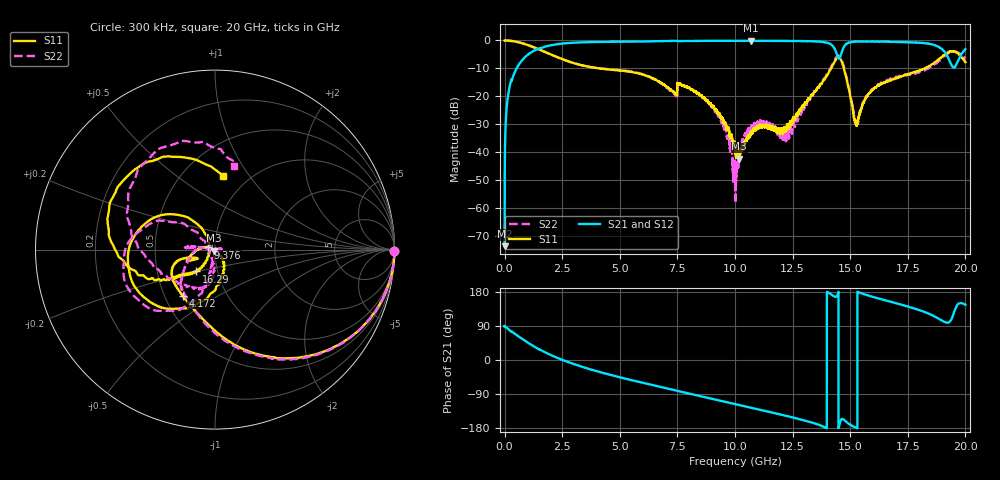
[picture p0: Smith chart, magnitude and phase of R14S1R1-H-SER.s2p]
!{R14S1R1}
!Johanson Technology Inc.
!www.johansontechnology.com
!Test Board Conditions:
!Substrate Type  RO4350B
!Substrate Thickness  20 mil
!Substrate Dk  3.66
!TL Type: GCPW
!TL Trace Width  36 mil
!TL Gap  12 mil
!Electrode orientation  Horizontal
!DUT TOPOLOGY	SERIES
!Mounting Pad LxW  26x36 mil
! Created Wed Nov 25 17:33:21 2020
! 2 Port Network Data from SP1.SP block
! freq  magS11  angS11  magS21  angS21  magS12  angS12  magS22  angS22
# khz S ma R 50
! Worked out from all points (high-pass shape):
!   20001 points, 300 kHz to 20 GHz, reference 50 ohm
!   highest |S21| = -0.11 dB at 10.7 GHz (marker M1); lowest = -73.7 dB at 300 kHz (marker M2)
!   |S21| within 3 dB of the highest: 1.418 GHz to 14.33 GHz (12.92 GHz wide, 164 % of centre); 14.68 GHz to 18.99 GHz (4.305 GHz wide, 25.6 % of centre)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
!   lowest |S11| = -42.4 dB at 10.19 GHz (marker M3), VSWR 1.02, Z = 49.5 - j0.603 ohm
!   |S11| at or under -10 dB: 4.107949 GHz to 4.109791 GHz (1.842 MHz wide, 0.0448 % of centre); 4.111 GHz to 14.17 GHz (10.06 GHz wide, 110 % of centre); 14.73 GHz to 18.24 GHz (3.514 GHz wide, 21.3 % of centre)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
!   |S22| runs from -57.4 to 0.0 dB; largest |S21 - S12| = 0.014
!   S11 on the Smith chart (normalised r, x): 300 kHz: open; 4.172 GHz: 0.62, -0.35; 9.376 GHz: 0.92, +0.02; 16.29 GHz: 0.79, -0.20; 20 GHz: 0.78, +0.76
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300  0.9968 -0.4  0.0002076 89.2  0.0002318 83.9  0.9983 -0.3
136300  0.9951 -6.8  0.09369 82.9  0.09427 82.9  0.9948 -6.8
524300  0.9462 -23.6  0.3174 65.8  0.3179 65.9  0.9453 -23.9
1944300  0.5772 -74.1  0.8086 14.9  0.8098 14.9  0.5735 -75.6
3334300  0.3609 -107.2  0.9241 -17.4  0.9243 -17.4  0.3597 -107.6
4172300  0.3133 -125.2  0.9414 -32.5  0.9416 -32.5  0.3155 -119.8
6667300  0.1866 -164.1  0.9714 -69.6  0.9724 -69.6  0.1839 -152.5
9376300  0.04201 163.5  0.985 -107.6  0.9852 -107.7  0.03806 171.3
1.00003e7  0.01298 -179.6  0.9847 -116.3  0.9861 -116.3  0.004202 126.7
1.01863e7  0.007617 -127.0  0.9844 -118.8  0.983 -118.8  0.01069 12.9
1.06973e7  0.023 -86.1  0.9871 -125.9  0.9828 -125.8  0.02892 1.4
1.22693e7  0.02997 -57.8  0.9792 -148.1  0.9797 -148.1  0.02414 -60.0
1.33343e7  0.1062 -61.5  0.9663 -165.2  0.9669 -165.2  0.1061 -99.9
1.40503e7  0.2559 -97.2  0.8957 177.8  0.9008 177.6  0.2676 -109.2
1.44723e7  0.4957 -159.6  0.4953 175.8  0.4976 175.6  0.5315 -156.8
1.47253e7  0.3176 141.7  0.7639 -157.5  0.764 -157.6  0.3401 151.6
1.52683e7  0.03001 -176.2  0.9533 -178.9  0.9541 -179.0  0.03463 -155.2
1.62913e7  0.161 -131.0  0.9548 161.3  0.9525 161.3  0.1661 -96.5
1.66673e7  0.186 -136.2  0.9479 155.2  0.9437 155.2  0.1947 -100.8
1.85003e7  0.3597 -152.4  0.8598 119.7  0.8569 119.6  0.3352 -160.5
1.92743e7  0.6221 164.4  0.4673 99.1  0.474 99.1  0.5919 139.9
2e7  0.4088 83.2  0.6978 145.8  0.694 146.4  0.4718 77.1
